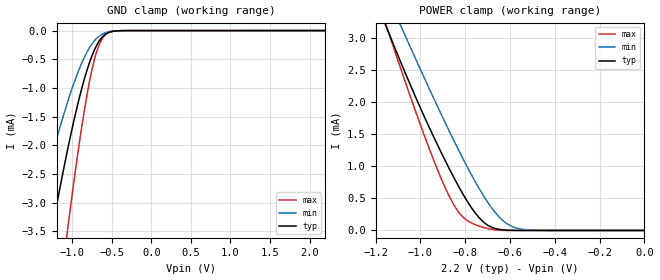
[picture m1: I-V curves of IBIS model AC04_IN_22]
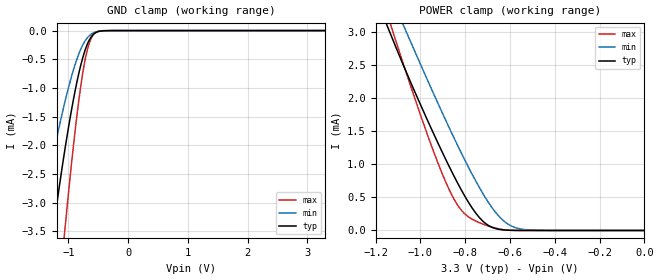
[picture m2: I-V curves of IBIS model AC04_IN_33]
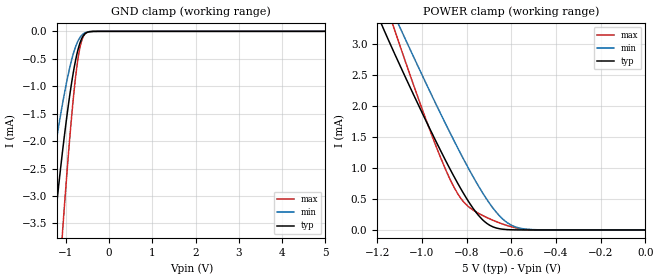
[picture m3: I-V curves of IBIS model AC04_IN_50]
| TEXAS INSTRUMENTS INCORPORATED
| Standard Linear and Logic Group
| IBIS Model of SN74AC04
| HEX INVRTERS
| This file contains package information for the following:
|  SOIC 14-pin (D) package as [Component] AC04_D
|  SSOP 14-pin (DB) package as [Component] AC04_DB
|  PDIP 14-pin (N) package as [Component] AC04_N
|  TSSOP 14-pin (PW) package as [Component] AC04_PW
| This device can be powered at the following Vccs:
|  2.2 volt Vcc
|  3.3 volt Vcc
|  5 volt Vcc
| This file provides unique models under the [Model Selector] for each Vcc.
| For operation at a specific Vcc, select the appropriate model after each
| [Model Selector] keyword.
[IBIS Ver]   3.2
[Comment char]  |_char
[File Name]   sn74ac04.ibs
[File Rev]   1.1 | a_die
[Date]   August 29, 2002
[Source]   Data created from TI-SPICE simulations at TI-SLL.
[Notes]   The following is an IBIS list for the AC04.
   Please contact sllibis@ti.com with questions and
   comments concerning SLL IBIS models.
   This IBIS model is created from a BA (back annotated netlist
[Disclaimer] Property of Texas Instruments Incorporated.  Unauthorized
   reproduction and/or distribution is strictly prohibited.
   This product is protected under copyright law.
   Created  2002, (C) Copyright  2002, Texas Instruments
   Incorporated, All Rights Reserved
   UNLESS THERE IS A SIGNED, WRITTEN AGREEMENT TO THE
   CONTRARY, TEXAS INSTRUMENTS (TI) IS PROVIDING THE IBIS
   MODELS  AND WITHOUT ANY WARRANTY, EXPRESSED OR
   IMPLIED.  TI assumes no liability for:
   1) the accuracy of the IBIS models provided to your
   company;
   2) the proper functioning of these IBIS Models in your
   design or for any resulting applications; or
   3) infringement of patents, copyrights or intellectual
   property rights resulting from your use of these IBIS
   models.
   TI provides IBIS Models as a service to our customers.
   You and your company shall not distribute, sell or give
   these models to anyone else without prior written
   permission from TI.
   TI reserves the right to make changes to our products or
   to discontinue any semiconductor product or service
   without notice, and advises our customers to obtain the
   latest version of relevant information to verify, before
   placing orders, that the information being relied on is
   current.
   Please be aware that your receipt and use of the IBIS
   information provided shall serve as acceptance of these
   terms and conditions.  If you do not accept these terms,
   you should return or destroy the IBIS models and any
   other accompanying information immediately.
| Component AC04_D 14-pin SOIC
[Component]   AC04_D
[Manufacturer]   Texas Instruments, Inc.
[Package]
|   typ   min   max
R_pkg   3.100e-02   2.800e-02   3.400e-02
L_pkg   3.109e-09   2.462e-09   3.889e-09
C_pkg   4.730e-13   3.630e-13   6.280e-13
[Pin]   signal_name   model_name   R_pin   L_pin   C_pin
1   1A   AC04_IN   3.300e-02   3.854e-09   6.220e-13
2   1Y   AC04_OUT   3.200e-02   3.188e-09   4.730e-13
3   2A   AC04_IN   2.800e-02   2.462e-09   3.770e-13
4   2Y   AC04_OUT   3.100e-02   2.596e-09   3.630e-13
5   3A   AC04_IN   2.800e-02   2.521e-09   3.720e-13
6   3Y   AC04_OUT   3.400e-02   3.250e-09   4.760e-13
7   GND   GND   3.400e-02   3.889e-09   6.280e-13
8   4Y   AC04_OUT   3.400e-02   3.889e-09   6.280e-13
9   4A   AC04_IN   3.400e-02   3.250e-09   4.760e-13
10   5Y   AC04_OUT   2.800e-02   2.521e-09   3.720e-13
11   5A   AC04_IN   3.100e-02   2.596e-09   3.640e-13
12   6Y   AC04_OUT   2.800e-02   2.462e-09   3.770e-13
13   6A   AC04_IN   3.200e-02   3.188e-09   4.730e-13
14   VCC   POWER   3.300e-02   3.854e-09   6.220e-13
| Component AC04_DB 14-pin SSOP
[Component]   AC04_DB
[Manufacturer]   Texas Instruments, Inc.
[Package]
|   typ   min   max
R_pkg   4.400e-02   4.100e-02   4.600e-02
L_pkg   3.551e-09   3.258e-09   3.927e-09
C_pkg   4.020e-13   3.600e-13   4.210e-13
[Pin]   signal_name   model_name   R_pin   L_pin   C_pin
1   1A   AC04_IN   4.600e-02   3.927e-09   4.080e-13
2   1Y   AC04_OUT   4.400e-02   3.587e-09   4.210e-13
3   2A   AC04_IN   4.100e-02   3.289e-09   3.980e-13
4   2Y   AC04_OUT   4.200e-02   3.258e-09   3.600e-13
5   3A   AC04_IN   4.100e-02   3.286e-09   4.030e-13
6   3Y   AC04_OUT   4.400e-02   3.586e-09   4.210e-13
7   GND   GND   4.600e-02   3.927e-09   4.080e-13
8   4Y   AC04_OUT   4.600e-02   3.927e-09   4.080e-13
9   4A   AC04_IN   4.400e-02   3.586e-09   4.210e-13
10   5Y   AC04_OUT   4.100e-02   3.286e-09   4.030e-13
11   5A   AC04_IN   4.300e-02   3.258e-09   3.600e-13
12   6Y   AC04_OUT   4.100e-02   3.289e-09   3.980e-13
13   6A   AC04_IN   4.400e-02   3.587e-09   4.210e-13
14   VCC   POWER   4.600e-02   3.927e-09   4.080e-13
| Component AC04_N 14-pin PDIP
[Component]   AC04_N
[Manufacturer]   Texas Instruments, Inc.
[Package]
|   typ   min   max
R_pkg   4.500e-02   3.700e-02   6.300e-02
L_pkg   5.407e-09   3.922e-09   6.942e-09
C_pkg   3.890e-13   2.050e-13   6.040e-13
[Pin]   signal_name   model_name   R_pin   L_pin   C_pin
1   1A   AC04_IN   6.300e-02   6.942e-09   6.040e-13
2   1Y   AC04_OUT   3.700e-02   6.200e-09   4.060e-13
3   2A   AC04_IN   4.200e-02   4.389e-09   3.220e-13
4   2Y   AC04_OUT   3.800e-02   3.922e-09   2.050e-13
5   3A   AC04_IN   3.900e-02   4.301e-09   2.980e-13
6   3Y   AC04_OUT   3.800e-02   5.329e-09   3.560e-13
7   GND   GND   5.300e-02   6.510e-09   5.440e-13
8   4Y   AC04_OUT   5.300e-02   6.437e-09   5.390e-13
9   4A   AC04_IN   3.900e-02   5.352e-09   3.470e-13
10   5Y   AC04_OUT   4.200e-02   4.473e-09   2.970e-13
11   5A   AC04_IN   4.400e-02   4.326e-09   2.250e-13
12   6Y   AC04_OUT   4.200e-02   4.295e-09   2.800e-13
13   6A   AC04_IN   4.200e-02   6.318e-09   4.180e-13
14   VCC   POWER   6.100e-02   6.900e-09   6.030e-13
| Component AC04_PW 14-pin TSSOP
[Component]   AC04_PW
[Manufacturer]   Texas Instruments, Inc.
[Package]
|   typ   min   max
R_pkg   3.200e-02   2.900e-02   3.500e-02
L_pkg   2.378e-09   2.170e-09   2.680e-09
C_pkg   3.140e-13   2.700e-13   3.350e-13
[Pin]   signal_name   model_name   R_pin   L_pin   C_pin
1   1A   AC04_IN   3.300e-02   2.618e-09   3.300e-13
2   1Y   AC04_OUT   3.100e-02   2.313e-09   3.170e-13
3   2A   AC04_IN   3.000e-02   2.310e-09   3.140e-13
4   2Y   AC04_OUT   3.100e-02   2.173e-09   2.720e-13
5   3A   AC04_IN   3.000e-02   2.204e-09   3.090e-13
6   3Y   AC04_OUT   3.200e-02   2.315e-09   3.170e-13
7   GND   GND   3.500e-02   2.680e-09   3.350e-13
8   4Y   AC04_OUT   3.300e-02   2.640e-09   3.330e-13
9   4A   AC04_IN   3.400e-02   2.347e-09   3.190e-13
10   5Y   AC04_OUT   2.900e-02   2.277e-09   3.130e-13
11   5A   AC04_IN   3.100e-02   2.170e-09   2.700e-13
12   6Y   AC04_OUT   3.100e-02   2.244e-09   3.110e-13
13   6A   AC04_IN   3.300e-02   2.343e-09   3.210e-13
14   VCC   POWER   3.500e-02   2.657e-09   3.320e-13
| Model AC04_IN
[Model Selector]   AC04_IN
AC04_IN_22   2.2 volt Vcc
AC04_IN_33   3.3 volt Vcc
AC04_IN_50   5 volt Vcc
| Model AC04_OUT
[Model Selector]   AC04_OUT
AC04_OUT_22   2.2 volt Vcc
AC04_OUT_33   3.3 volt Vcc
AC04_OUT_50   5 volt Vcc
| Models and submodels in the file (6): AC04_IN_22 (Input), AC04_IN_33 (Input), AC04_IN_50 (Input), AC04_OUT_22 (Output), AC04_OUT_33 (Output), AC04_OUT_50 (Output)
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[Model]   AC04_IN_22
Model_type  Input
Vinl = 0.7
Vinh = 1.56
| variable   typ   min   max
C_comp   1.04pF   0.93pF   1.44pF
[Temperature Range]   40   100   -40
| Ambient temperature   25   85   -40
[Voltage range]   2.2   2   2.4
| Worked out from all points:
|   GND clamp passes 1 mA (typ) near -0.88 V on its own axis
|   POWER clamp passes 1 mA (typ) near -0.88 V on its own axis
[GND Clamp]
| AC04_IN_22
|   Voltage   I(typ)   I(min)   I(max)
-5V       -46.92mA   -30.58mA   -59.62mA
-1.515V   -5.634mA   -3.566mA   -8.947mA
-1.465V   -5.197mA   -3.282mA   -8.307mA
-1.265V   -3.555mA   -2.213mA   -5.828mA
-1.065V   -2.109mA   -1.269mA   -3.528mA
-900mV    -1.111mA   -628.4uA   -1.852mA
-780mV    -547.1uA   -291.8uA   -867.5uA
-685mV    -239.6uA   -126.8uA   -337.8uA
-630mV    -126.3uA   -69.97uA   -160uA
-570mV    -53.62uA   -32.51uA   -58.58uA
-390mV    -2.065uA   -1.475uA   -1.141uA
2.2V      1.335nA    1.043nA    2.375nA
[POWER Clamp]
| AC04_IN_22
|   Voltage   I(typ)   I(min)   I(max)
-5V       45.66mA    43.34mA    48.79mA
-1.175V   3.374mA    3.881mA    3.433mA
-1.14V    3.068mA    3.602mA    3.064mA
-1.105V   2.768mA    3.326mA    2.699mA
-1.075V   2.516mA    3.091mA    2.392mA
-905mV    1.2mA      1.795mA    791.1uA
-845mV    788.2uA    1.362mA    367.6uA
-790mV    451.2uA    984.8uA    153.1uA
-695mV    72.51uA    417uA      26.97uA
-635mV    10.75uA    165.4uA    1.922uA
-575mV    1.278uA    41.58uA    48.79nA
-84.45fV  1.335nA    467.8pA    3.795nA
[Model]   AC04_IN_33
Model_type  Input
Vinl = 0.9
Vinh = 2.1
| variable   typ   min   max
C_comp   1.05pF   0.85pF   1.23pF
[Temperature Range]   40   100   -40
| Ambient temperature   25   85   -40
[Voltage range]   3.3   3   3.6
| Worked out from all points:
|   GND clamp passes 1 mA (typ) near -0.88 V on its own axis
|   POWER clamp passes 1 mA (typ) near -0.88 V on its own axis
[GND Clamp]
| AC04_IN_33
|   Voltage   I(typ)   I(min)   I(max)
-5V       -46.92mA   -30.58mA   -59.62mA
-1.51V    -5.59mA    -3.537mA   -8.882mA
-1.255V   -3.478mA   -2.163mA   -5.708mA
-1.065V   -2.109mA   -1.269mA   -3.528mA
-895mV    -1.084mA   -611.8uA   -1.806mA
-835mV    -784.3uA   -429.3uA   -1.285mA
-770mV    -508.4uA   -270.1uA   -799.3uA
-720mV    -336.7uA   -177uA     -500.7uA
-670mV    -203.9uA   -108.8uA   -280uA
-560mV    -45.8uA    -28.19uA   -48.68uA
-405mV    -2.787uA   -1.951uA   -1.676uA
3.3V      4.213nA    12.06nA    20.26nA
[POWER Clamp]
| AC04_IN_33
|   Voltage   I(typ)   I(min)   I(max)
-5V       45.66mA    43.87mA    49.1mA
-1.145V   3.061mA    3.64mA     3.232mA
-1.11V    2.769mA    3.364mA    2.864mA
-1.075V   2.485mA    3.09mA     2.501mA
-1.04V    2.208mA    2.818mA    2.144mA
-890mV    1.094mA    1.685mA    756.1uA
-840mV    755.6uA    1.327mA    415uA
-785mV    423.5uA    951.8uA    204.9uA
-695mV    72.52uA    417uA      64.94uA
-630mV    9.041uA    150.1uA    12.41uA
-575mV    1.283uA    41.58uA    638.1nA
-84.45fV  4.213nA    632.2pA    31.47nA
[Model]   AC04_IN_50
Model_type  Input
Vinl = 1.65
Vinh = 3.85
| variable   typ   min   max
C_comp   1.10pF   0.93pF   1.71pF
[Temperature Range]   40   100   -40
| Ambient temperature   25   85   -40
[Voltage range]   5   4.5   5.5
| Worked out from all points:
|   GND clamp passes 1 mA (typ) near -0.88 V on its own axis
|   POWER clamp passes 1 mA (typ) near -0.88 V on its own axis
[GND Clamp]
| AC04_IN_50
|   Voltage   I(typ)   I(min)   I(max)
-5V       -46.92mA   -30.58mA   -59.62mA
-1.56V    -6.035mA   -3.826mA   -9.528mA
-1.51V    -5.59mA    -3.537mA   -8.882mA
-1.305V   -3.869mA   -2.418mA   -6.312mA
-1.255V   -3.478mA   -2.163mA   -5.708mA
-1.08V    -2.21mA    -1.334mA   -3.692mA
-1.06V    -2.076mA   -1.247mA   -3.474mA
-900mV    -1.111mA   -628.4uA   -1.852mA
-770mV    -508.4uA   -270.1uA   -799.3uA
-670mV    -203.9uA   -108.8uA   -280.1uA
-550mV    -38.99uA   -24.34uA   -40.29uA
5V        16.38nA    4.859uA    150.6nA
[POWER Clamp]
| AC04_IN_50
|   Voltage   I(typ)   I(min)   I(max)
-5V       45.74mA    45.24mA    49.64mA
-1.17V    3.235mA    3.838mA    3.746mA
-1.125V   2.87mA     3.482mA    3.262mA
-1.075V   2.477mA    3.09mA     2.732mA
-965mV    1.638mA    2.244mA    1.62mA
-895mV    1.129mA    1.722mA    985.3uA
-840mV    755.6uA    1.327mA    587.5uA
-785mV    423.6uA    951.8uA    357.6uA
-695mV    72.53uA    417uA      176.8uA
-640mV    12.79uA    181.6uA    97.2uA
-585mV    1.851uA    53.91uA    37.94uA
-84.45fV  16.38nA    947.5pA    229.7nA
